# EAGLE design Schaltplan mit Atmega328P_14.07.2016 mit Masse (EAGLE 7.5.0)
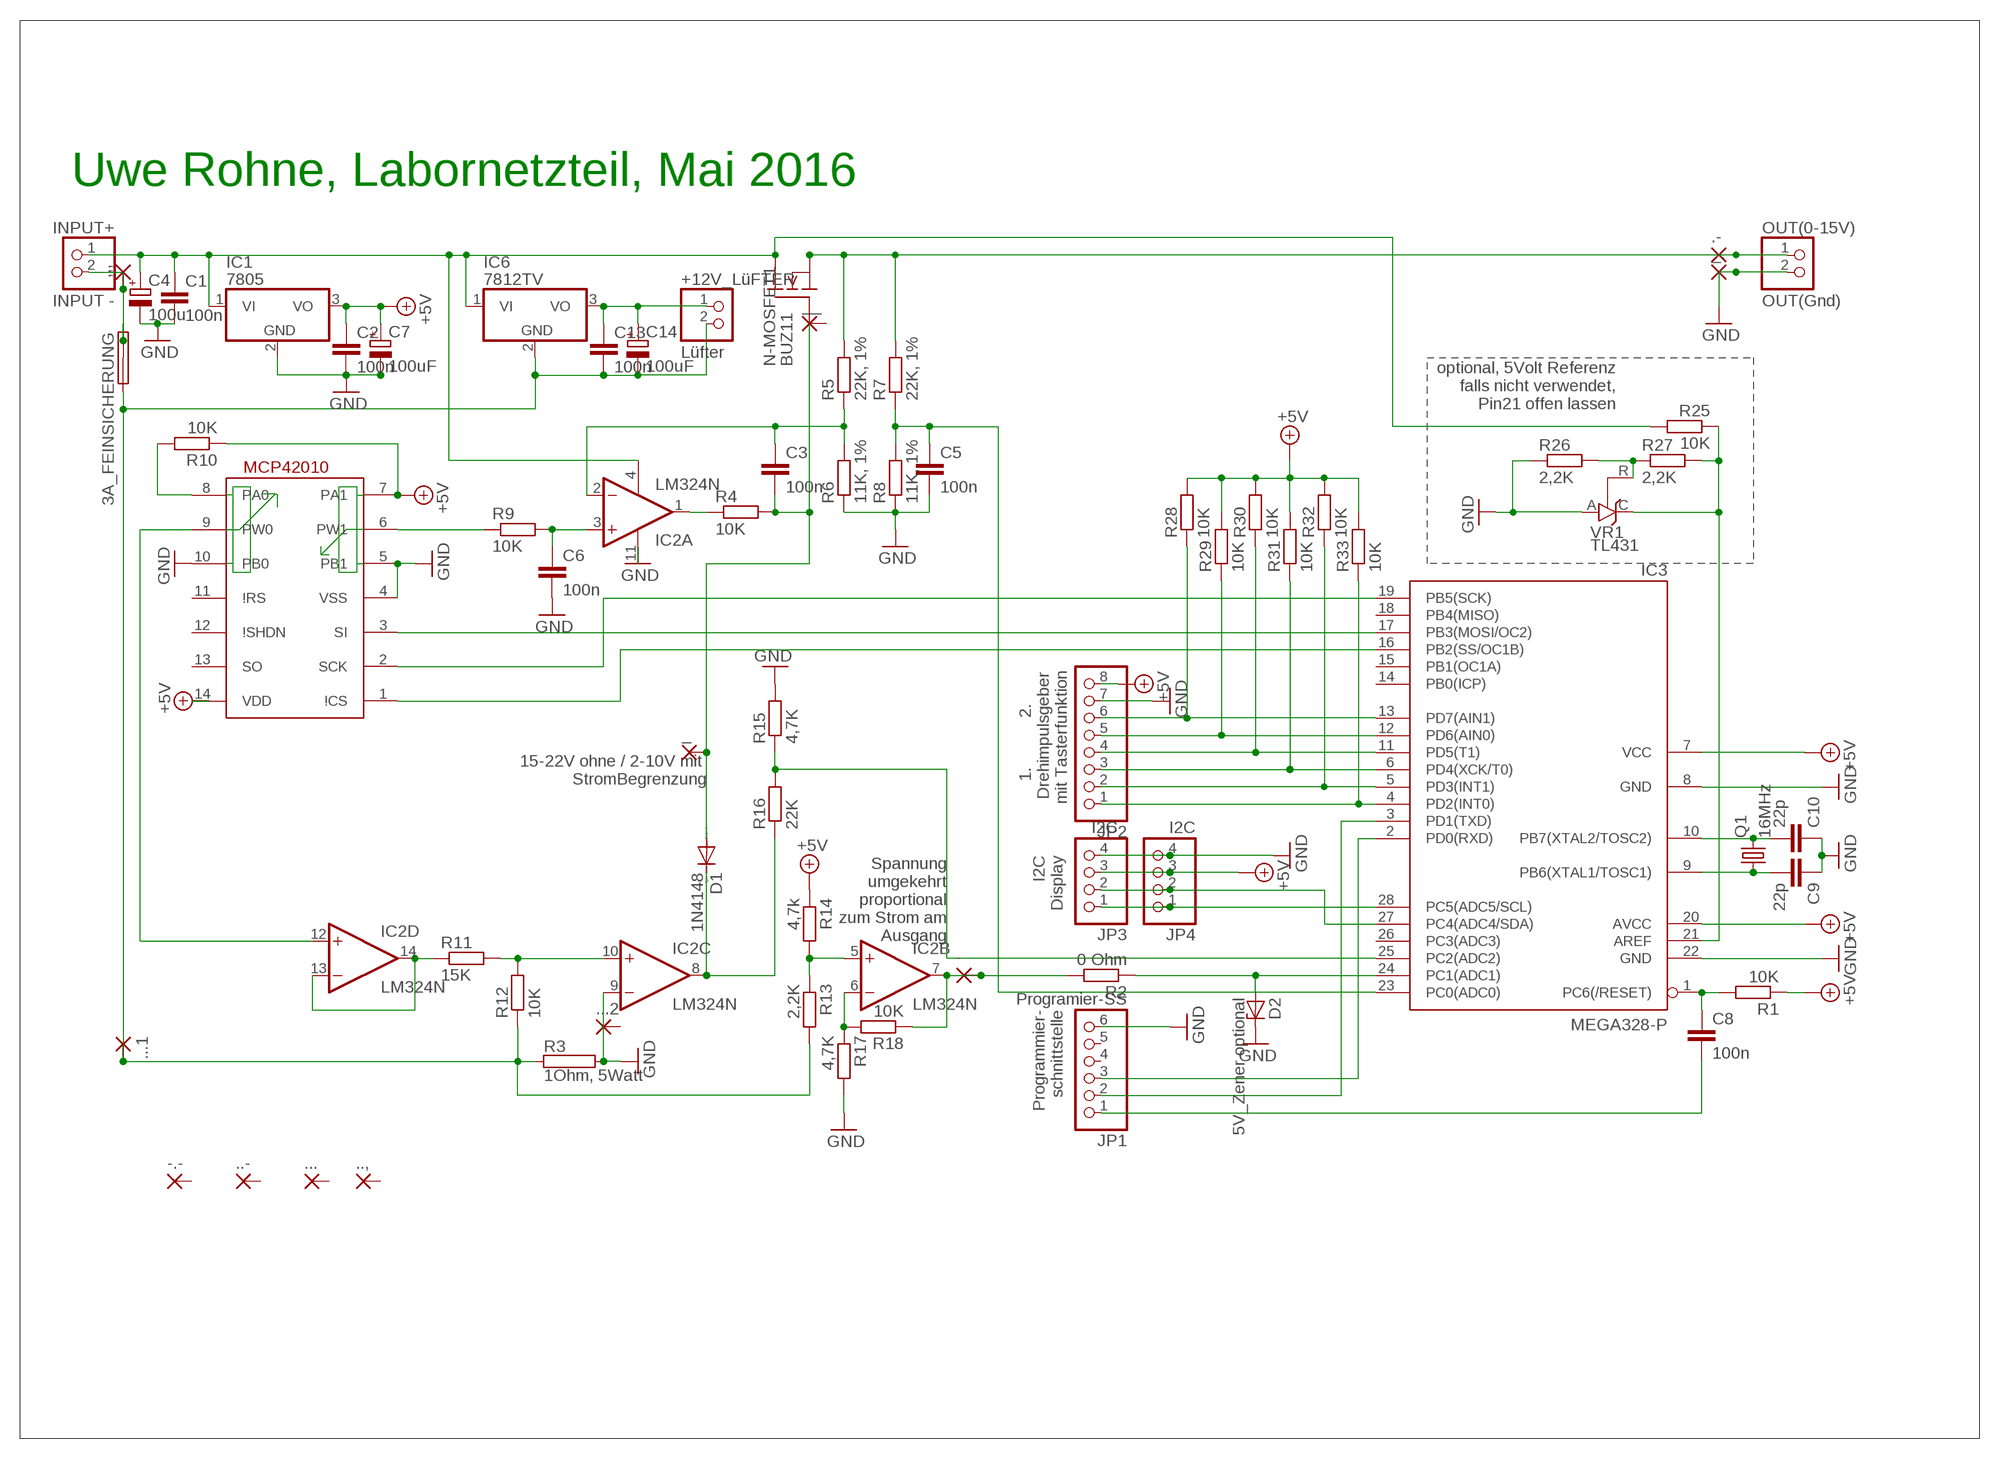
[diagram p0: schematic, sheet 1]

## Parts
3A_FEINSICHERUNG  SHK20L  [SHK20L]
+12V_LüFTER  Lüfter  PINHD-1X2  [1X02]
,,,  2,54/1,0  [2,54/1,0]
-  2,54/0,8  [2,54/0,8]
-.-  2,54/1,0  [2,54/1,0]
.-  2,54/1,0  [2,54/1,0]
..,  2,54/1,0  [2,54/1,0]
..-  2,54/1,0  [2,54/1,0]
...  2,54/1,0  [2,54/1,0]
...1  2,54/1,0  [2,54/1,0]
...2  2,54/1,0  [2,54/1,0]
_  2,54/0,8  [2,54/0,8]
_.  2,54/1,0  [2,54/1,0]
__  2,54/1,0  [2,54/1,0]
C1  100n  C-EU075-063X106  [C075-063X106]
C2  100n  C-EU075-063X106  [C075-063X106]
C3  100n  C-EU075-063X106  [C075-063X106]
C4  100u  CPOL-EUE15-6AXIAL  [E15-6]
C5  100n  C-EU075-063X106  [C075-063X106]
C6  100n  C-EU075-063X106  [C075-063X106]
C7  100uF  CPOL-EUE15-6AXIAL  [E15-6]
C8  100n  C-EU075-063X106  [C075-063X106]
C9  22p  C-EU075-063X106  [C075-063X106]
C10  22p  C-EU075-063X106  [C075-063X106]
C13  100n  C-EU075-063X106  [C075-063X106]
C14  100uF  CPOL-EUE15-6AXIAL  [E15-6]
D1  1N4148  1N4148DO35-7  [DO35-7]
D2  5V_Zener optional  ZENER-DIODEZD-5  [ZDIO-5]
IC1  7805  7805T  [TO220H]
IC2  LM324N  [DIL14]
IC3  MEGA328-P  MEGA8-P  [DIL28-3]
IC6  7812TV  [TO220V]
INPUT+  INPUT -  PINHD-1X2  [1X02]
JP1  Programier-SS  PINHD-1X6  [1X06]
JP2  PINHD-1X8  [1X08]
JP3  I2C  PINHD-1X4  [1X04]
JP4  I2C  PINHD-1X4  [1X04]
N-MOSFET1  BUZ11  [TO220]
OUT(0-15V)  OUT(Gnd)  PINHD-1X2  [1X02]
Q1  16MHz  CRYSTALHC18U-V  [HC18U-V]
R1  10K  R-EU_0204/7  [0204/7]
R2  0 Ohm  R-EU_0204/7  [0204/7]
R3  1Ohm, 5Watt  RAC01  [AC01]
R4  10K  R-EU_0204/7  [0204/7]
R5  22K, 1%  R-EU_0204/7  [0204/7]
R6  11K, 1%  R-EU_0204/7  [0204/7]
R7  22K, 1%  R-EU_0204/7  [0204/7]
R8  11K, 1%  R-EU_0204/7  [0204/7]
R9  10K  R-EU_0204/7  [0204/7]
R10  10K  R-EU_0204/7  [0204/7]
R11  15K  R-EU_0204/7  [0204/7]
R12  10K  R-EU_0204/7  [0204/7]
R13  2,2K  R-EU_0204/7  [0204/7]
R14  4,7k  R-EU_0204/7  [0204/7]
R15  4,7K  R-EU_0204/7  [0204/7]
R16  22K  R-EU_0204/7  [0204/7]
R17  4,7K  R-EU_0204/7  [0204/7]
R18  10K  R-EU_0204/7  [0204/7]
R25  10K  R-EU_0204/7  [0204/7]
R26  2,2K  R-EU_0204/7  [0204/7]
R27  2,2K  R-EU_0204/7  [0204/7]
R28  10K  R-EU_0207/2V  [0207/2V]
R29  10K  R-EU_0207/2V  [0207/2V]
R30  10K  R-EU_0207/2V  [0207/2V]
R31  10K  R-EU_0207/2V  [0207/2V]
R32  10K  R-EU_0207/2V  [0207/2V]
R33  10K  R-EU_0207/2V  [0207/2V]
U$5  MCP42010-I/P  [DIL-14]
VR1  TL431  TL431CLP  [TO92-CLP]

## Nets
7812: C1.1 C4.+ IC1.1(VI) IC2.4(P:V+) IC6.1(VI) INPUT+.1 N-MOSFET1.2(D) R25.2
+5V: C2.1 C7.+ IC1.3(VO) IC3.7(VCC) IC3.20(AVCC) JP2.8 JP3.3 JP4.3 R1.1 R10.1 R14.1 R28.2 R29.2 R30.2 R31.2 R32.2 R33.2 U$5.7(PA1) U$5.14(VDD)
GND: _..1(P) C1.2 C2.2 C4.- C5.2 C6.2 C7.- C9.1 C10.1 D2.C IC1.2(GND) IC2.9(C:-IN) IC2.11(P:V-) IC3.8(GND) IC3.22(GND) JP1.6 JP2.7 JP3.4 JP4.4 OUT(0-15V).2 R3.2 R6.1 R8.1 R15.2 R17.2 R26.1 U$5.4(VSS) U$5.5(PB1) U$5.10(PB0) VR1.A
N$1: C5.1 IC3.23(PC0(ADC0)) R7.1 R8.2
N$2: IC3.19(PB5(SCK)) U$5.2(SCK)
N$3: IC3.17(PB3(MOSI/OC2)) U$5.3(SI)
N$4: IC3.16(PB2(SS/OC1B)) U$5.1(\!CS)
N$5: C10.2 IC3.10(PB7(XTAL2/TOSC2)) Q1.2
N$6: C9.2 IC3.9(PB6(XTAL1/TOSC1)) Q1.1
N$7: IC3.28(PC5(ADC5/SCL)) JP3.1 JP4.1
N$8: IC3.21(AREF) R25.1 R27.2 VR1.C
N$9: IC3.4(PD2(INT0)) JP2.1 R33.1
N$10: IC3.27(PC4(ADC4/SDA)) JP3.2 JP4.2
N$11: IC3.2(PD0(RXD)) JP1.3
N$12: IC3.5(PD3(INT1)) JP2.2 R32.1
N$13: IC3.6(PD4(XCK/T0)) JP2.3 R31.1
N$14: IC3.11(PD5(T1)) JP2.4 R30.1
N$15: +12V_LüFTER.1 C13.1 C14.+ IC6.3(VO)
N$16: IC2.1(A:OUT) R4.1
N$17: D2.A IC3.24(PC1(ADC1)) R2.1
N$18: IC2.5(B:+IN) R13.1 R14.2
N$19: C3.1 IC2.2(A:-IN) R5.1 R6.2
N$20: .-.1(P) N-MOSFET1.3(S) OUT(0-15V).1 R5.2 R7.2
N$21: R9.1 U$5.6(PW1)
N$22: C6.1 IC2.3(A:+IN) R9.2
N$23: IC2.12(D:+IN) U$5.9(PW0)
N$24: IC2.13(D:-IN) IC2.14(D:OUT) R11.1
N$25: R10.2 U$5.8(PA0)
N$26: IC2.10(C:+IN) R11.2 R12.2
N$27: 3A_FEINSICHERUNG.1A 3A_FEINSICHERUNG.1B ,,,.1(P) INPUT+.2
N$28: IC2.6(B:-IN) R17.1 R18.2
N$29: IC3.25(PC2(ADC2)) R15.1 R16.2
N$30: -.1(P) IC2.7(B:OUT) R2.2 R18.1
N$31: C8.1 IC3.1(PC6(/RESET)) R1.2
N$32: R26.2 R27.1 VR1.R
N$33: IC3.12(PD6(AIN0)) JP2.5 R29.1
N$34: C8.2 JP1.1
N$35: D1.C IC2.8(C:OUT) R16.1
N$36: IC3.3(PD1(TXD)) JP1.2
N$37: IC3.13(PD7(AIN1)) JP2.6 R28.1
N$43: 3A_FEINSICHERUNG.2A +12V_LüFTER.2 ...1.1(P) C13.2 C14.- IC6.2(GND) R3.1 R12.1 R13.2
N$45: _.1(P) C3.2 D1.A N-MOSFET1.1(G) R4.2
Unconnected: 3A_FEINSICHERUNG.2B -.-.1(P) ..,.1(P) ..-.1(P) ...2.1(P) ....1(P) __.1(P) IC3.14(PB0(ICP)) IC3.15(PB1(OC1A)) IC3.18(PB4(MISO)) IC3.26(PC3(ADC3)) JP1.4 JP1.5 U$5.11(\!RS) U$5.12(\!SHDN) U$5.13(SO)

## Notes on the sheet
- Uwe Rohne, Labornetzteil, Mai 2016
- optional, 5Volt Referenz
  falls nicht verwendet,
  Pin21 offen lassen
- 15-22V ohne / 2-10V mit 
  StromBegrenzung
- 1.           2.
   Drehimpulsgeber
  mit Tasterfunktion
- I2C
  Display
- Spannung
  umgekehrt
  proportional
  zum Strom am
  Ausgang
- Programmier-
  schnittstelle

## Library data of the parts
3A_FEINSICHERUNG = fuse:SHK20L: FUSE HOLDER 5 x 20 mm, SH contact, SHH1 Schukat, E1073 Buerklin; OC_FARNELL: unknown; OC_NEWARK: unknown
+12V_LüFTER INPUT+ OUT(0-15V) = pinhead:PINHD-1X2: PIN HEADER
,,, -.- .- .., ..- ... ...1 ...2 _. __ = wirepad:2,54/1,0: THROUGH-HOLE PAD
- _ = wirepad:2,54/0,8: THROUGH-HOLE PAD
C1-C3 C5 C6 C8-C10 C13 = resistor:C-EU: CAPACITOR, European symbol
C4 C7 C14 = rcl:CPOL-EU: POLARIZED CAPACITOR, European symbol
D1 = diode:1N4148: DIODE
D2 = diode:ZENER-DIODE: Z-Diode
IC1 IC6 = linear:78*: Positive VOLTAGE REGULATOR Source: http://cache.national.com/ds/LM/LM78L05.pdf http://www.fairchildsemi.com/ds/LM/LM7805.pdf
IC2 = linear:LM324: OP AMP
IC3 = atmel:MEGA8-P: MICROCONTROLLER 8 Kbytes FLASH, 1 kbytes SRAM, 512 bytes EEPROM, USART, 4-channel 10 bit ADC, 2-channel 8 bit ADC Pin compatible with Atmega48, ATMega88, ATMega168 Source: avr.lbr; OC_FARNELL: unknown; OC_NEWARK: unknown
JP1 = pinhead:PINHD-1X6: PIN HEADER
JP2 = pinhead:PINHD-1X8: PIN HEADER
JP3 JP4 = pinhead:PINHD-1X4: PIN HEADER
N-MOSFET1 = transistor-fet:BUZ11: N-Channel Enhancement MOSFET 50V; 30A; 0,040Ohm
Q1 = crystal:CRYSTAL: CRYSTAL; OC_FARNELL: unknown; OC_NEWARK: unknown
R1 R2 R4-R18 R25-R33 = rcl:R-EU_: RESISTOR, European symbol
R3 = resistor-power:R: Power Resitor; OC_FARNELL: unknown; OC_NEWARK: unknown
U$5 = dig-pot:MCP42010-I/P
VR1 = v-reg:TL431CLP: VOLTAGE REGULATOR

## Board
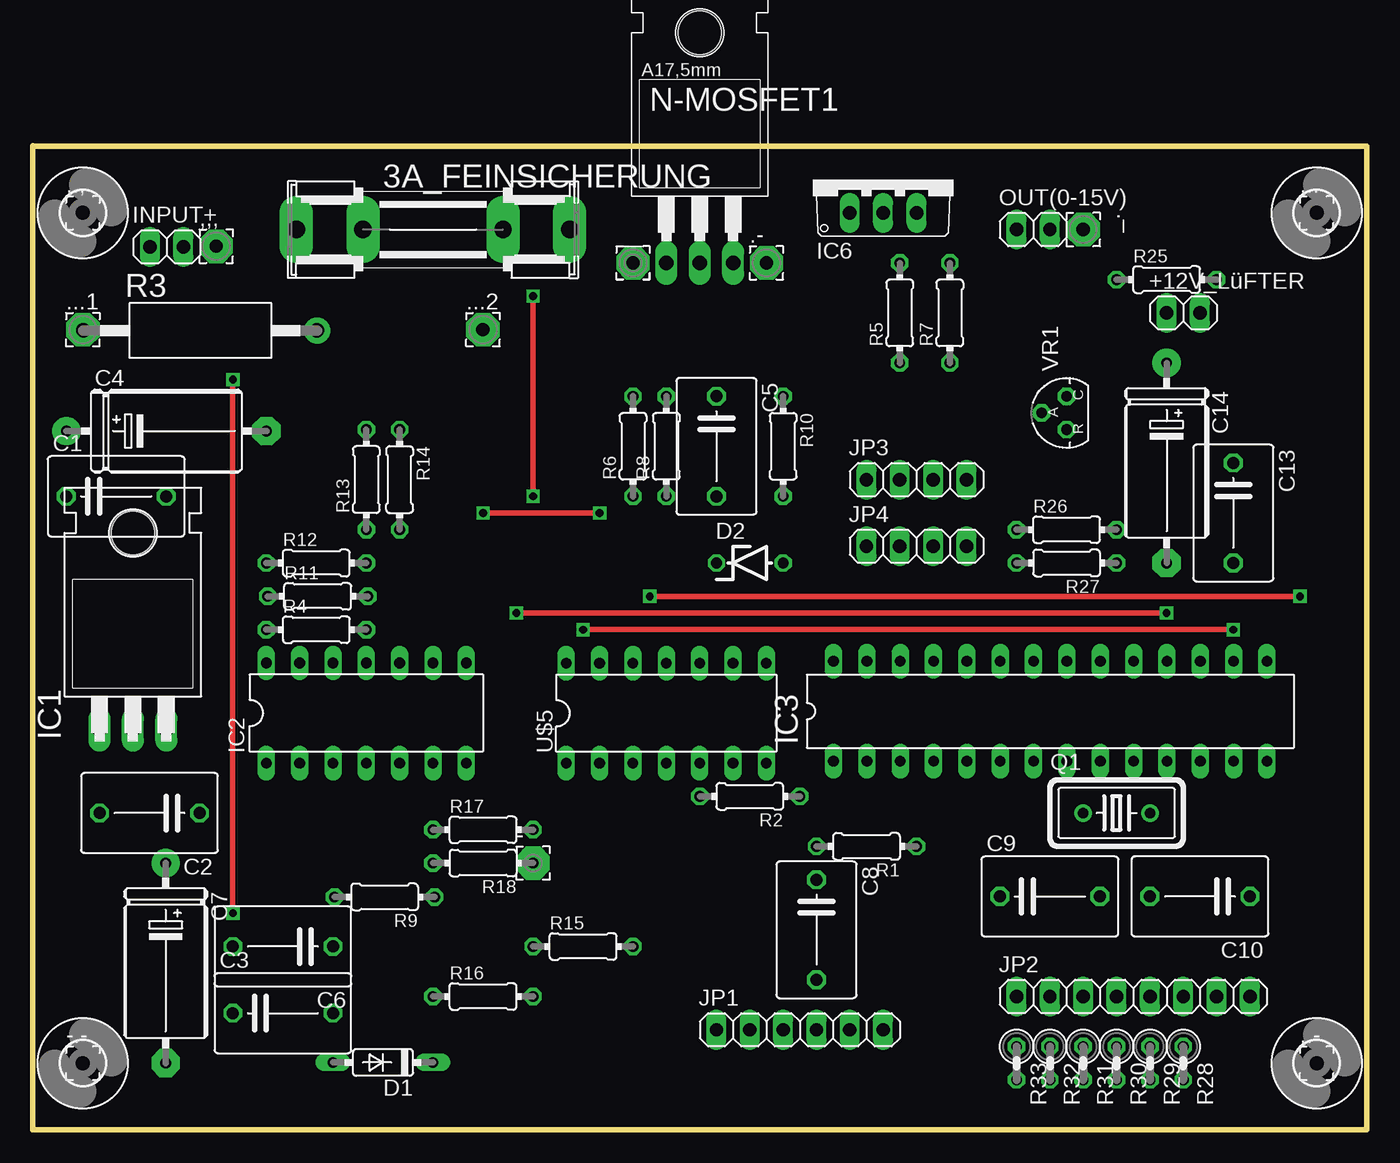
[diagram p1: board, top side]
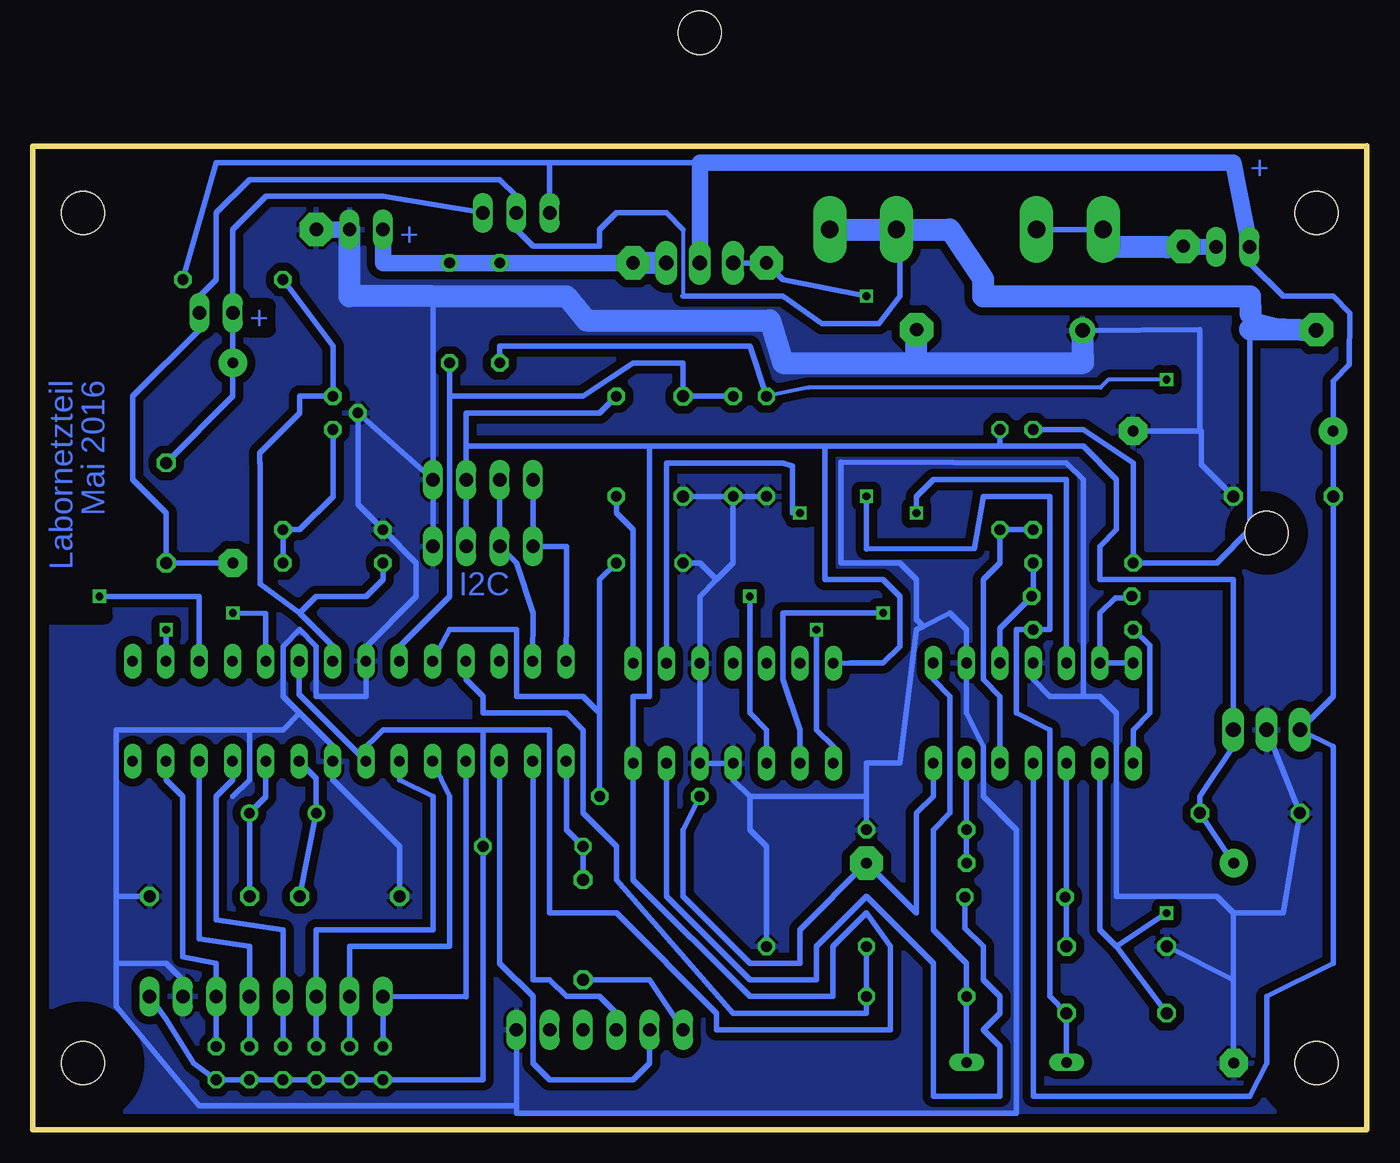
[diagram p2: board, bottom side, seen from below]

Size 101.6 x 74.96 mm. Coordinates in mm from the lower left corner, seen from the top.
Outline: 101.6,74.93 0,74.96 0,74.93
Outline: 0,74.93 101.6,74.93
Outline: 101.6,74.93 101.6,0 0,0 0,74.93
Copper layers (1*16): Top 0.035mm / dielectric 1.5mm / Bottom 0.035mm
Design rules "default": minimum track width 10mil, minimum drill 24mil, track to track 8mil, track to pad 8mil, pad to pad 8mil, via to via 8mil, smd to smd 8mil, copper to edge 40mil, drill to drill 8mil, minimum pad ring 10mil, minimum via ring 8mil, stop-mask expansion 4mil, vias tented up to drill 0mil, thermal gap 10mil

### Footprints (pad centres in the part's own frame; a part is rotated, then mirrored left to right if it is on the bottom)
SHK20L = drill 1.321 pad 2.54 long: 1A -10.414,0; 1B -5.334,0; 2A 10.414,0; 2B 5.334,0
1X02 = drill 1.016 long: 1 -1.27,0; 2 1.27,0
2,54/1,0 = drill 1.016 pad 2.54 octagon: 1 0,0
2,54/0,8 = drill 0.813 pad 2.54 octagon: 1 0,0
C075-063X106 = drill 0.914 octagon: 1 -3.81,0; 2 3.81,0
E15-6 = drill 0.813 pad 2.159: + -7.62,0 | drill 0.813 pad 2.159 octagon: - 7.62,0
DO35-7 = drill 0.813 long: A 3.81,0; C -3.81,0
ZDIO-5 = drill 0.813 octagon: A 2.54,0; C -2.54,0
TO220H = drill 1.118 long: 1 -2.54,-10.16; 2 0,-10.16; 3 2.54,-10.16 | hole 3.302: 0,4.826
DIL14 = drill 0.813 long: 1 -7.62,-3.81; 2 -5.08,-3.81; 3 -2.54,-3.81; 4 0,-3.81; 5 2.54,-3.81; 6 5.08,-3.81; 7 7.62,-3.81; 8 7.62,3.81; 9 5.08,3.81; 10 2.54,3.81; 11 0,3.81; 12 -2.54,3.81; 13 -5.08,3.81; 14 -7.62,3.81
DIL28-3 = drill 0.813 long: 1 -16.51,-3.81; 2 -13.97,-3.81; 3 -11.43,-3.81; 4 -8.89,-3.81; 5 -6.35,-3.81; 6 -3.81,-3.81; 7 -1.27,-3.81; 8 1.27,-3.81; 9 3.81,-3.81; 10 6.35,-3.81; 11 8.89,-3.81; 12 11.43,-3.81; 13 13.97,-3.81; 14 16.51,-3.81; 15 16.51,3.81; 16 13.97,3.81; 17 11.43,3.81; 18 8.89,3.81; 19 6.35,3.81; 20 3.81,3.81; 21 1.27,3.81; 22 -1.27,3.81; 23 -3.81,3.81; 24 -6.35,3.81; 25 -8.89,3.81; 26 -11.43,3.81; 27 -13.97,3.81; 28 -16.51,3.81
TO220V = drill 1.016 long: 1 -2.54,-2.54; 2 0,-2.54; 3 2.54,-2.54
1X06 = drill 1.016 long: 1 -6.35,0; 2 -3.81,0; 3 -1.27,0; 4 1.27,0; 5 3.81,0; 6 6.35,0
1X08 = drill 1.016 long: 1 -8.89,0; 2 -6.35,0; 3 -3.81,0; 4 -1.27,0; 5 1.27,0; 6 3.81,0; 7 6.35,0; 8 8.89,0
1X04 = drill 1.016 long: 1 -3.81,0; 2 -1.27,0; 3 1.27,0; 4 3.81,0
TO220 = drill 1.118 long: 1 -2.54,-6.35; 2 0,-6.35; 3 2.54,-6.35 | hole 3.302: 0,11.176
HC18U-V = drill 0.813: 1 -2.54,0; 2 2.54,0
0204/7 = drill 0.813 octagon: 1 -3.81,0; 2 3.81,0
AC01 = drill 1.1 pad 2: 1 -8.9,0; 2 8.9,0
0207/2V = drill 0.813 octagon: 1 -1.27,0; 2 1.27,0
3,3 = hole 3.3: 0,0
DIL-14 = drill 0.813 long: 1 -7.62,-3.81; 2 -5.08,-3.81; 3 -2.54,-3.81; 4 0,-3.81; 5 2.54,-3.81; 6 5.08,-3.81; 7 7.62,-3.81; 8 7.62,3.81; 9 5.08,3.81; 10 2.54,3.81; 11 0,3.81; 12 -2.54,3.81; 13 -5.08,3.81; 14 -7.62,3.81
TO92-CLP = drill 0.813 octagon: A 0,1.905; C 1.27,0; R -1.27,0

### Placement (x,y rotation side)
3A_FEINSICHERUNG  30.48,68.58 0 top
+12V_LüFTER  87.63,62.23 0 top
,,,  13.97,67.31 0 top
-  38.1,20.32 0 top
-.-  3.81,5.08 0 top
.-  55.88,66.04 0 top
..,  3.81,69.85 0 top
..-  97.79,5.08 0 top
...  97.79,69.85 0 top
...1  3.81,60.96 0 top
...2  34.29,60.96 0 top
_  45.72,66.04 0 top
_.  80.01,68.58 270 top
__  45.72,66.04 0 top
C1  6.35,48.26 0 top
C2  8.89,24.13 180 top
C3  19.05,8.89 0 top
C4  10.18,53.23 0 top
C5  52.07,52.07 270 top
C6  19.05,13.97 180 top
C7  10.12,12.7 270 top
C8  59.69,15.24 270 top
C9  77.47,17.78 0 top
C10  88.9,17.78 180 top
C13  91.44,46.99 270 top
C14  86.36,50.8 270 top
D1  26.67,5.13 180 top
D2  54.61,43.18 0 top
IC1  7.62,40.64 0 top
IC2  25.4,31.75 0 top
IC3  77.5,31.89 0 top
IC6  64.77,72.39 0 top
INPUT+  10.2,67.26 0 top
JP1  58.42,7.62 0 top
JP2  83.82,10.16 0 top
JP3  67.31,49.53 0 top
JP4  67.31,44.45 0 top
N-MOSFET1  50.8,72.39 0 top
OUT(0-15V)  76.2,68.58 0 top
Q1  82.55,24.13 0 top
R1  63.5,21.59 180 top
R2  54.61,25.4 180 top
R3  12.75,60.88 0 top
R4  21.59,38.1 0 top
R5  66.04,62.23 90 top
R6  45.72,52.07 90 top
R7  69.85,62.23 90 top
R8  48.26,52.07 90 top
R9  26.79,17.74 180 top
R10  57.15,52.07 270 top
R11  21.7,40.64 0 top
R12  21.59,43.18 0 top
R13  25.4,49.53 90 top
R14  27.94,49.53 270 top
R15  41.91,13.97 0 top
R16  34.29,10.16 0 top
R17  34.29,22.86 0 top
R18  34.29,20.32 180 top
R25  86.36,64.77 0 top
R26  78.74,45.72 0 top
R27  78.74,43.18 180 top
R28  87.63,5.08 270 top
R29  85.09,5.08 270 top
R30  82.55,5.08 270 top
R31  80.01,5.08 270 top
R32  77.47,5.08 270 top
R33  74.93,5.08 270 top
U$1  [3,3]  3.81,5.08 0 top
U$2  [3,3]  97.79,5.08 0 top
U$3  [3,3]  97.79,69.85 0 top
U$4  [3,3]  3.81,69.85 0 top
U$5  48.25,31.73 0 top
VR1  78.74,54.61 90 top

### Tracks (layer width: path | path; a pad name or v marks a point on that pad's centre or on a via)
7812
  Bottom 0.406: 8.89,67.26 INPUT+.1 8.89,66.04 6.35,63.5 2.54,63.5 1.27,62.23 1.31,58.31 2.54,57.04 | 2.54,57.04 C4.+ 2.56,48.26 | 2.54,57.04 2.54,54.61 | 2.56,48.26 2.56,33 IC1.1 2.54,29.21 2.54,12.7 7.62,10.16 7.62,5.08 8.89,2.54 25.4,2.54 IC2.4 | C1.1 2.56,48.26 | 62.23,73.66 87.63,73.66 R25.2 | 62.23,73.66 IC6.1 | 50.8,73.66 62.23,73.66
  Bottom 1.27: 8.89,67.26 10.16,73.66 50.8,73.66 N-MOSFET1.2
+5V
  Bottom 0.406: U$5.14 39.36,35.55 36.83,35.56 35.56,36.83 35.56,40.64 36.83,41.91 41.27,41.91 41.27,52.07 | IC3.20 81.31,33.16 76.78,28.63 | 76.78,28.63 IC3.7 | 67.31,30.48 62.23,30.48 62.23,16.51 57.15,16.51 49.53,8.89 49.53,7.62 36.27,7.62 36.27,13.97 38.1,16.51 40.64,13.97 40.64,10.16 46.99,10.16 55.88,19.05 U$5.7 55.88,33.02 54.61,33.02 54.61,52.07 | 67.31,30.48 74.93,30.48 76.78,28.63 | 27.94,52.07 41.27,52.07 | 41.27,52.07 54.61,52.07 | JP2.8 91.44,8.43 89.36,5.08 R28.2 R29.2 R30.2 R31.2 R32.2 R33.2 67.31,3.81 R1.1 67.31,30.48 | C7.+ 10.16,20.32 C2.1 12.7,25.4 10.16,29.21 IC1.3 10.16,41.91 20.32,41.91 20.32,44.45 19.05,45.72 19.05,49.53 21.59,52.07 27.94,52.07 | R10.1 58.42,54.61 68.58,54.61 68.58,52.07 | R14.1 27.94,52.07 | 68.58,52.07 JP3.3 JP4.3 | 54.61,52.07 68.58,52.07
GND
  Bottom 0.406: IC1.2 C2.2 6.35,16.51 10.16,16.51 | U$5.10 50.8,35.56 | U$5.10 50.79,36.82 50.8,36.83 | 85.09,30.48 82.55,30.48 81.28,31.75 | 85.09,30.48 95.25,30.48 95.25,17.78 | 81.28,31.75 78.77,29.24 IC3.8 78.77,26.7 73.66,21.59 C9.1 | 81.28,31.75 82.55,33.02 82.55,36.83 81.28,38.1 80.01,36.83 80.01,33.02 76.2,33.02 76.2,35.67 IC3.22 76.23,36.8 72.39,40.64 72.39,43.18 R26.1 76.83,47.62 VR1.A JP3.4 | U$5.10 U$5.5 U$5.4 48.26,26.67 46.99,25.4 | R17.2 38.1,25.4 | U$5.10 | 33.78,38.35 31.75,39.37 30.48,38.1 IC2.9 30.48,31.75 29.21,29.21 29.21,25.4 26.67,22.86 26.67,1.27 64.77,1.27 64.77,1.83 | 33.78,38.35 34.29,38.1 35.56,27.94 38.1,27.94 38.1,25.4 | IC2.11 25.4,34.29 24.13,33.02 21.59,33.02 | 21.59,33.02 20.32,33.02 19.05,31.75 19.05,17.78 11.43,17.78 10.16,16.51 | 38.1,25.4 46.99,25.4 | JP1.6 64.77,1.83 | 64.77,1.83 88.92,1.83 95.25,9.42 95.25,12.7 | 49.53,41.91 48.26,43.18 R8.1 | 49.53,41.91 50.8,40.64 50.79,40.63 U$5.10 | 95.25,12.7 95.25,17.78 | C4.- 12.7,53.23 | 12.7,53.23 12.59,53.23 12.59,50.69 C1.2 | 86.36,25.4 85.09,26.67 85.09,30.48 | R15.2 45.72,21.59 46.99,22.86 46.99,25.4 | C6.2 10.16,11.43 | 10.16,11.43 10.16,5.12 C7.- | 10.16,16.51 10.16,11.43 | 21.59,33.02 21.59,49.53 22.86,50.8 40.06,50.85 40.06,43.18 35.56,43.18 34.29,41.91 34.29,38.86 33.78,38.35 | JP3.4 71.12,63.5 | R3.2 12.7,60.96 12.7,53.23 | R8.1 R6.1 | R8.1 C5.2 | D2.C 50.8,43.18 49.53,41.91 | JP4.4 JP3.4 | C10.1 95.25,17.78 | JP2.7 90.17,11.43 91.44,12.7 95.25,12.7
  Bottom 1.27: OUT(0-15V).2 _..1
  Bottom 1.676: OUT(0-15V).2 77.47,63.5 71.12,63.5 60.96,63.5 59.44,61.65 45.47,61.65 44.45,58.42 34.29,58.42 | 34.29,58.42 21.59,58.42 R3.2 | 34.29,58.42 34.29,60.96
  pour Bottom (isolate 0.61): -2.54,77.47 109.22,77.47 109.22,76.2 106.68,76.2 106.68,-1.27 -8.89,-1.27 -8.89,0 -2.54,0
N$1
  Bottom 0.406: IC3.23 73.69,36.8 69.85,40.64 69.85,55.88 | 69.85,55.88 R7.1 | 69.85,55.88 59.69,55.88 55.88,58.42 52.07,58.42 C5.1 R8.2
N$2  (via drill 0.6)
  Top 0.406: v86.36,39.37 v36.83,39.37
  Bottom 0.406: U$5.2 43.17,30.47 44.45,34.29 44.45,39.37 v36.83,39.37 | IC3.19 83.85,39.34 v86.36,39.37
N$3  (via drill 0.6)
  Top 0.406: v96.52,40.64 v46.99,40.64
  Bottom 0.406: IC3.17 88.93,40.61 v96.52,40.64 | v46.99,40.64 46.99,31.75 45.72,30.48 U$5.3
N$4  (via drill 0.6)
  Top 0.406: v41.91,38.1 v91.44,38.1
  Bottom 0.406: U$5.1 40.63,29.2 41.91,30.48 v41.91,38.1 | v91.44,38.1 91.44,35.73 IC3.16
N$5
  Bottom 0.406: IC3.10 83.85,25.37 Q1.2 C10.2
N$6
  Bottom 0.406: IC3.9 80.01,26.78 Q1.1 C9.2
N$7
  Bottom 0.406: 60.96,35.73 IC3.28 60.96,39.37 60.96,44.45 JP4.1 JP3.1
N$8
  Bottom 0.406: 81.28,39.37 84.3,41.58 84.3,50.77 84.33,50.8 84.33,51.56 81.28,54.61 81.28,55.88 VR1.C 78.74,59.69 R25.1 | 81.28,39.37 78.74,36.83 78.74,35.73 IC3.21 | R27.2 74.93,41.91 76.2,40.64 80.01,40.64 81.28,39.37
N$9
  Bottom 0.406: R33.1 JP2.1 68.61,10.13 IC3.4
N$10
  Bottom 0.406: IC3.27 63.5,39.37 64.77,43.18 JP4.2 JP3.2
N$11
  Bottom 0.406: IC3.2 63.5,28.05 63.5,11.43 62.23,11.43 60.96,10.16 58.42,10.16 57.15,8.89 JP1.3
N$12
  Bottom 0.406: R32.1 JP2.2 77.47,13.97 69.85,13.97 69.85,25.4 IC3.5
N$13
  Bottom 0.406: R31.1 JP2.3 80.01,15.24 71.12,15.24 71.12,25.4 73.66,26.67 IC3.6
N$14
  Bottom 0.406: R30.1 JP2.4 82.55,15.24 87.63,16 87.63,25.4 86.36,26.67 86.36,28.05 IC3.11
N$15
  Bottom 0.406: C13.1 86.36,55.88 C14.+ +12V_LüFTER.1 86.36,68.58 83.82,71.12 74.93,71.12 IC6.3
N$16
  Bottom 0.406: R4.1 16.51,36.88 16.51,31.75 17.78,30.48 IC2.1
N$17
  Bottom 0.406: R2.1 58.42,31.75 | 58.42,31.75 59.69,33.02 64.77,33.02 64.77,38.1 69.85,38.1 IC3.24 | D2.A 58.42,41.91 58.42,31.75
N$18
  Bottom 0.406: IC2.5 27.94,33.02 29.21,34.29 29.21,41.91 27.94,43.18 R14.2 R13.1
N$19  (via drill 0.6)
  Top 0.406: v15.24,57.15 v15.24,16.51
  Bottom 0.305: v15.24,57.15 19.66,57.15 20.27,56.54 42.52,56.54 R6.2
  Bottom 0.406: C3.1 19.05,13.97 | 19.05,13.97 20.32,15.24 IC2.2 | v15.24,16.51 19.05,13.97 | R6.2 46.99,59.69 66.04,59.69 R5.1
N$20
  Bottom 1.27: .-.1 R5.2 R7.2 74.93,66.04 OUT(0-15V).1
  Bottom 1.676: N-MOSFET1.3 .-.1
N$21
  Bottom 0.406: U$5.6 53.34,17.78 46.99,11.43 41.91,11.43 41.91,13.97 38.1,17.78 33.02,12.7 33.02,2.54 27.94,2.54 27.94,6.35 29.21,7.62 27.94,8.89 27.94,10.16 29.21,11.43 29.21,13.97 30.6,15.36 R9.1
N$22
  Bottom 0.406: IC2.3 22.86,17.62 | 22.86,17.62 R9.2 | 22.86,17.62 C6.1
N$23  (via drill 0.6)
  Top 0.406: v34.29,46.99 v43.18,46.99
  Bottom 0.406: U$5.9 53.34,50.8 44.45,50.8 43.74,50.57 43.74,46.99 v43.18,46.99 | IC2.12 22.86,49.53 33.02,49.53 34.29,48.26 v34.29,46.99
N$24
  Bottom 0.406: R11.1 17.78,40.53 19.16,40.53 20.32,39.37 IC2.13 IC2.14
N$25
  Bottom 0.406: U$5.8 55.88,45.72 57.15,46.99 R10.2
N$26
  Bottom 0.406: 25.51,43.07 R12.2 25.4,40.75 R11.2 27.94,38.21 IC2.10
N$27
  Bottom 0.406: INPUT+.2 11.52,67.31 ,,,.1 | 3A_FEINSICHERUNG.1A 3A_FEINSICHERUNG.1B
  Bottom 1.27: INPUT+.2 15.2,67.23
  Bottom 1.676: 15.2,67.23 20.07,67.23 3A_FEINSICHERUNG.1A
N$28
  Bottom 0.406: IC2.6 R17.1 R18.2
N$29
  Bottom 0.406: IC3.25 68.61,34.32 67.31,33.02 67.31,31.75 60.96,31.75 59.69,30.48 59.69,24.13 57.15,21.59 57.15,19.05 48.26,8.89 38.1,8.89 R16.2 R15.1
N$30
  Bottom 0.406: IC2.7 33.02,25.4 34.29,24.13 34.29,16.51 -.1 43.18,15.24 43.18,12.7 46.99,12.7 52.07,17.78 52.07,22.86 R2.2
N$31
  Bottom 0.406: IC3.1 60.96,28.05 60.96,22.86 R1.2 C8.1
N$32
  Bottom 0.406: R27.1 R26.2 81.28,45.72 78.74,48.26 VR1.R
N$33
  Bottom 0.406: R29.1 JP2.5 85.09,13.97 88.93,14.53 IC3.12
N$34
  Bottom 0.406: JP1.1 54.61,11.43 C8.2
N$35
  Bottom 0.406: D1.C R16.1 30.48,12.7 33.02,15.24 33.02,22.86 31.75,24.13 31.75,33.02 33.02,34.29 IC2.8
N$36
  Bottom 0.406: 66.04,28.11 IC3.3 66.04,28.05 66.04,12.7 63.5,10.16 63.5,5.08 62.23,3.81 55.88,3.81 54.61,5.08 JP1.2
N$37
  Bottom 0.406: IC3.13 91.44,28.05 91.44,26.67 90.17,25.4 90.17,13.18 87.63,12.7 JP2.6 R28.1
N$43
  Bottom 0.305: 52.07,68.58 52.07,63.5
  Bottom 0.406: C14.- C13.2 91.44,46.99 93.98,49.53 93.98,55.88 88.9,60.96 +12V_LüFTER.2 88.9,63.5 87.63,64.77 87.63,69.85 85.09,72.39 66.04,72.39 64.77,71.12 IC6.2 64.77,68.58 63.5,67.31 58.42,67.31 58.42,68.58 57.15,69.85 53.34,69.85 52.07,68.58 | R3.1 8.85,62.15 8.89,60.84 8.89,45.72 11.43,43.18 R12.1 17.78,50.8 21.59,53.34 R13.2 | 52.07,63.5 44.45,63.5 41.48,61.42 37.13,61.42 35.56,63.5 35.56,68.58
  Bottom 1.676: 8.85,62.15 8.89,63.5 29.21,63.5 29.21,64.77 31.75,68.58 35.56,68.58 3A_FEINSICHERUNG.2A | 8.89,60.96 6.35,60.96 R3.1 3.85,60.96 ...1.1
N$45  (via drill 0.6)
  Top 0.406: v38.1,48.26 v38.1,63.5
  Bottom 0.406: N-MOSFET1.1 _.1 44.45,64.77 v38.1,63.5 | D1.A C3.2 24.13,10.16 24.13,30.48 26.67,31.75 26.67,38.1 R4.2 24.13,38.1 24.13,48.26 29.21,48.26 29.87,44.27 38.1,44.25 v38.1,48.26

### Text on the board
Bottom: + | + | + | Labornetzteil / Mai 2016 | I2C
